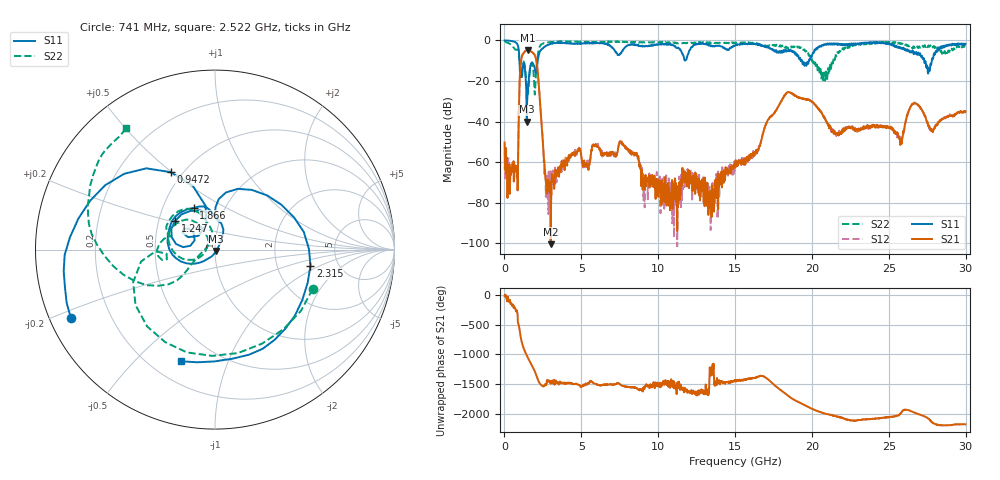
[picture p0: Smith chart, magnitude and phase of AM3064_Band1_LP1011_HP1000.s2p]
# Hz S DB R 50.0
!freq dBS11 angS11 dBS21 angS21 dBS12 angS12 dBS22 angS22
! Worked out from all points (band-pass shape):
!   1600 points, 10 MHz to 29.98 GHz, reference 50 ohm
!   highest |S21| = -4.67 dB at 1.51 GHz (marker M1); lowest = -100.5 dB at 3.009 GHz (marker M2)
!   |S21| within 3 dB of the highest: 1.144 GHz to 1.996 GHz (851.1 MHz wide, 54.2 % of centre)
!   lowest |S11| = -40.1 dB at 1.453 GHz (marker M3), VSWR 1.02, Z = 50.6 - j0.81 ohm
!   |S11| at or under -10 dB: 973.9 MHz to 2.162 GHz (1.188 GHz wide, 75.8 % of centre); 19.35 GHz to 19.81 GHz (453.3 MHz wide, 2.32 % of centre); 27.3 GHz to 27.8 GHz (496.1 MHz wide, 1.8 % of centre)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
!   |S22| runs from -26.7 to -0.3 dB; largest |S21 - S12| = 0.0067
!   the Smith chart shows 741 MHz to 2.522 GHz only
!   S11 on the Smith chart (normalised r, x): 741 MHz: 0.06, -0.22; 947.2 MHz: 0.43, +0.50; 1.247 GHz: 0.61, +0.21; 1.866 GHz: 0.71, +0.36; 2.315 GHz: 3.12, -0.79; 2.522 GHz: 0.32, -0.69
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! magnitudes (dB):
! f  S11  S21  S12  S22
! 10 MHz  0.0  -50.4  -56.1  -0.3
! 741 MHz  -1.0  -64.3  -62.7  -4.6
! 947.2 MHz  -6.1  -32.1  -32.0  -7.6
! 1.247 GHz  -11.3  -6.3  -6.2  -10.4
! 1.453 GHz  -40.1  -4.8  -4.7  -21.5
! 1.51 GHz  -26.4  -4.7  -4.6  -26.3
! 1.866 GHz  -11.7  -6.2  -6.2  -13.7
! 2.315 GHz  -5.4  -30.7  -30.6  -2.7
! 2.522 GHz  -3.7  -52.4  -52.9  -1.5
! 3.009 GHz  -1.7  -100.5  -74.0  -0.8
! 5.015 GHz  -1.5  -57.7  -57.7  -0.7
! 7.601 GHz  -6.0  -50.2  -51.0  -0.7
! 10 GHz  -2.0  -77.1  -72.8  -1.0
! 13.39 GHz  -2.7  -74.3  -78.1  -1.3
! 15 GHz  -2.6  -60.7  -61.3  -1.4
! 18.34 GHz  -5.5  -26.0  -26.0  -3.5
! 19.99 GHz  -8.0  -30.2  -30.2  -9.3
! 21.62 GHz  -1.5  -46.1  -46.5  -7.4
! 25 GHz  -1.4  -42.6  -42.9  -1.0
! 26.68 GHz  -5.8  -30.9  -30.8  -3.7
! 27.56 GHz  -16.4  -42.1  -41.7  -2.7
! 29.98 GHz  -1.7  -35.0  -35.6  -3.1
